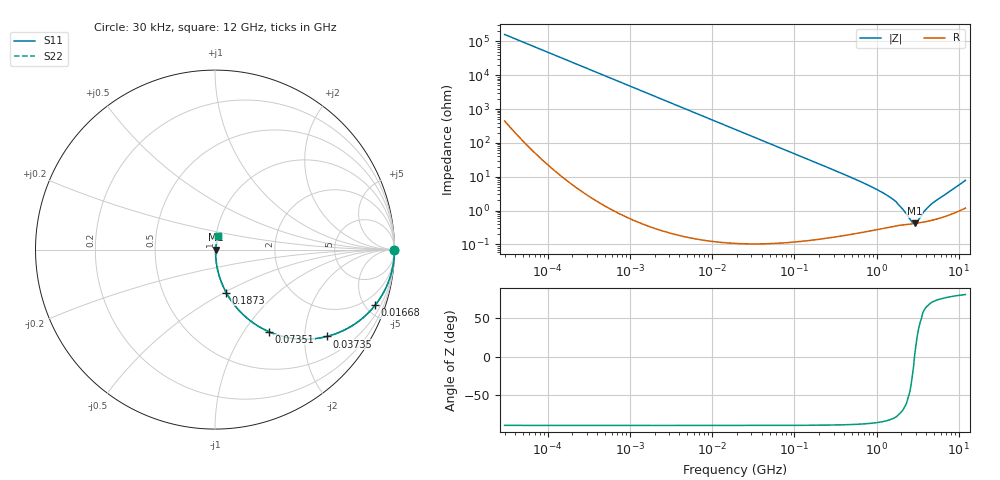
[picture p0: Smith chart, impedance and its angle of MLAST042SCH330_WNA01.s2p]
! MLAST042SCH330_WNA01  S-PARAMETER MODEL  ( General Type )
! Model Generated by TAIYO YUDEN Corporation (http://www.ty-top.com)
! Version 1.0
! TAIYO YUDEN Control No. 150820
! Copyright(c) 2015 TAIYO YUDEN CO.,LTD. All Rights Reserved.
! Product Description (link to TY-COMPAS)
! https://ds.yuden.co.jp/TYCOMPAS/or/detail?pn=MLAST042SCH330JWNA01&u=M
! Products Name : Multilayer Ceramic Capacitors
! Characteristics :
!  Capacitance : 33 pF , Rated Voltage : 25V , TCC : CH / C0H
!  Case Size : 0.4 x 0.2 / 0.016 x 0.008 [mm/inch] , Thickness : 0.2 / 0.008 [mm/inch]
!  (Conditions: Temperature = 25 degC , DC Bias Current/Voltage = 0A / 0V)
! External Node Assignments :
!  1  o---| |---o  2
! GND o---------o GND
! Frequency Range : 0.03MHz  -  12000MHz  [ 401 STEP ]
# MHz S RI R 50
! Freq[MHz].  S11 Real  S11 Imag  S21 Real  S21 Imag  S12 Real  S12 Imag  S22 Real  S22 Imag
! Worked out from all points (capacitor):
!   401 points, 30 kHz to 12 GHz, reference 50 ohm
!   read as one part in series: C = 33.1 pF near 32 kHz
!   lowest |Z| = 415 mohm at 2.904 GHz (marker M1)
!   series resonance near 2.888 GHz, so ESL is about 92 pH
!   S11 on the Smith chart (normalised r, x): 30 kHz: open; 16.68 MHz: 1.00, -5.77; 37.35 MHz: 1.00, -2.58; 73.51 MHz: 1.00, -1.31; 187.3 MHz: 1.00, -0.51; 12 GHz: 1.02, +0.15
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0.03  1 -0.000623  2.12e-06 0.000623  2.12e-06 0.000623  1 -0.000623
0.260295  1 -0.00541  3.03e-05 0.00541  3.03e-05 0.00541  1 -0.00541
2.258455  0.9978 -0.0468  0.0022 0.0468  0.0022 0.0468  0.9978 -0.0468
6.760619  0.9806 -0.1378  0.0194 0.1378  0.0194 0.1378  0.9806 -0.1378
16.67749  0.8927 -0.3093  0.1073 0.3093  0.1073 0.3093  0.8927 -0.3093
18.97367  0.8654 -0.3411  0.1346 0.3411  0.1346 0.3411  0.8654 -0.3411
37.34732  0.624 -0.484  0.376 0.484  0.376 0.484  0.624 -0.484
51.55976  0.4655 -0.4982  0.5345 0.4982  0.5345 0.4982  0.4655 -0.4982
73.51358  0.3 -0.4574  0.7 0.4574  0.7 0.4574  0.3 -0.4574
108.2504  0.1653 -0.3701  0.8347 0.3701  0.8347 0.3701  0.1653 -0.3701
164.6252  0.0793 -0.2679  0.9207 0.2679  0.9207 0.2679  0.0793 -0.2679
187.291  0.0626 -0.2395  0.9374 0.2395  0.9374 0.2395  0.0626 -0.2395
702.6322  0.00641 -0.0639  0.9936 0.0639  0.9936 0.0639  0.00641 -0.0639
1428.372  0.00384 -0.0252  0.9962 0.0252  0.9962 0.0252  0.00384 -0.0252
1790.1  0.00383 -0.0159  0.9962 0.0159  0.9962 0.0159  0.00383 -0.0159
2172.242  0.00386 -0.00873  0.9961 0.00873  0.9961 0.00873  0.00386 -0.00873
2635.962  0.00401 -0.00282  0.996 0.00282  0.996 0.00282  0.00401 -0.00282
2903.719  0.00413 0.000194  0.9959 -0.000194  0.9959 -0.000194  0.00413 0.000194
3097.169  0.00423 0.00195  0.9958 -0.00195  0.9958 -0.00195  0.00423 0.00195
3881.513  0.00472 0.00895  0.9953 -0.00895  0.9953 -0.00895  0.00472 0.00895
4864.487  0.0055 0.0161  0.9945 -0.0161  0.9945 -0.0161  0.0055 0.0161
12000  0.0174 0.0751  0.9826 -0.0751  0.9826 -0.0751  0.0174 0.0751
